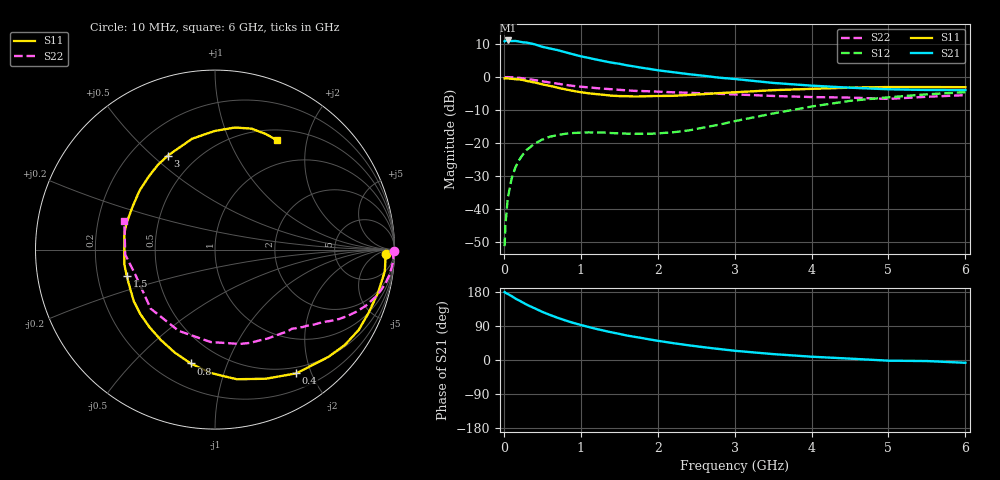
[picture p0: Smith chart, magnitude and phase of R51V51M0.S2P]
! SIEMENS Small Signal Semiconductors
! BFR183
! Si NPN RF Bipolar Junction Transistor in SOT23
! VCE = 1.5 V  IC = 1 mA
! Common Emitter S-Parameters:  May  1996
# GHz  S  MA  R  50
!  f  S11  S21  S12  S22
! GHz  MAG  ANG  MAG  ANG  MAG  ANG  MAG  ANG
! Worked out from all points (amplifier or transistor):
!   36 points, 10 MHz to 6 GHz, reference 50 ohm
!   highest |S21| = 11.1 dB at 50 MHz (marker M1)
!   |S21| within 3 dB of that: start of sweep to 709.4 MHz
!   unconditionally stable (mu >= 1): 1.628 GHz to 3.023 GHz
!   at 250 MHz: K = 0.16, MSG = 17.0 dB, |S12| = -23.5 dB
!   at 1.4 GHz: K = 0.86, MSG = 10.7 dB, |S12| = -17.0 dB
!   at 6 GHz: K = 0.97, MSG = 0.3 dB, |S12| = -4.6 dB
!   S11 on the Smith chart (normalised r, x): 10 MHz: 31, -16; 400 MHz: 0.41, -1.78; 800 MHz: 0.34, -0.75; 1.5 GHz: 0.33, -0.13; 3 GHz: 0.35, +0.56; 6 GHz: 0.63, +1.52
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0.01  0.9513 -1.5  3.489 179.3  0.0027 88.8  0.9986 -0.5
0.02  0.951 -3.0  3.553 177.6  0.0056 91.6  0.9893 -1.1
0.05  0.9539 -7.3  3.587 174.3  0.0141 85.2  0.9957 -2.9
0.1  0.9395 -14.8  3.509 168.9  0.0285 81.1  0.9901 -5.6
0.15  0.9257 -22.3  3.53 162.2  0.0423 76.8  0.9809 -8.5
0.3  0.87 -43.4  3.325 145.7  0.0786 64.6  0.9373 -15.9
0.4  0.825 -56.7  3.139 136.5  0.0971 57.5  0.8978 -20.3
0.5  0.7733 -68.5  2.875 127.0  0.1123 51.4  0.8606 -23.7
0.6  0.7324 -80.5  2.708 118.9  0.1241 46.0  0.8256 -26.6
0.7  0.6873 -92.1  2.557 111.3  0.1316 41.5  0.7925 -29.2
0.8  0.6486 -102.1  2.375 104.4  0.1375 37.6  0.7594 -31.5
0.9  0.6154 -111.5  2.212 98.1  0.141 34.8  0.7326 -33.3
1.1  0.5659 -130.1  1.952 87.2  0.1444 30.4  0.6951 -36.8
1.3  0.5363 -147.5  1.742 77.5  0.1433 28.2  0.6637 -39.8
1.5  0.5133 -163.1  1.589 69.0  0.1394 28.6  0.638 -42.8
1.7  0.5052 -178.4  1.442 61.1  0.137 31.1  0.6151 -45.8
2.2  0.5178 152.4  1.184 44.5  0.1447 41.6  0.586 -54.8
3  0.5857 116.8  0.933 24.4  0.2134 53.6  0.5438 -75.2
3.5  0.631 101.6  0.813 15.6  0.2793 52.1  0.5156 -92.7
4.5  0.6892 80.7  0.688 3.6  0.434 39.0  0.4865 -137.5
5.5  0.7034 66.2  0.635 -2.8  0.5455 22.1  0.501 -176.8
6  0.7003 60.7  0.632 -7.4  0.5881 12.2  0.5302 162.3
